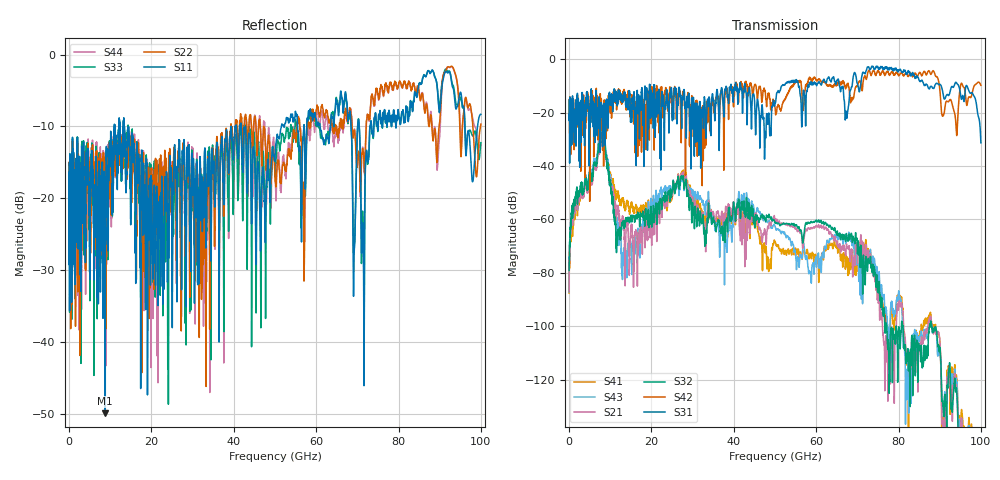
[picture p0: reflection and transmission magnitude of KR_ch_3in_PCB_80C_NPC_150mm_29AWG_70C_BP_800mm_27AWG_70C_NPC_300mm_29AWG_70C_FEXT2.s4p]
# GHz S RI R 45
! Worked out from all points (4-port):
!   4000 points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, 25 MHz to 100 GHz, reference 45 ohm
!   strongest paths, dB at 25 MHz, 25.02 GHz, 50.02 GHz, 75.03 GHz, 100 GHz:
!     S31: -20.7, -17.6, -16.4, -3.0, -31.3
!     S42: -20.7, -17.7, -18.0, -4.4, -9.7
!     S32: -79.1, -49.5, -61.3, -84.9, -155.0
!     S21: -86.8, -50.4, -60.1, -87.8, -157.8
!     S43: -87.1, -48.6, -62.6, -81.2, -149.6
!     S41: -87.6, -51.8, -68.5, -83.1, -149.4
!   lowest |S11| = -50.0 dB at 8.8 GHz (marker M1), VSWR 1.01, Z = 44.8 - j0.241 ohm
!   |S11| at or under -10 dB: start of sweep to 11.02 GHz; 13.41 GHz to 39.39 GHz (25.99 GHz wide, 98.4 % of centre); 42.84 GHz to 51.56 GHz (8.725 GHz wide, 18.5 % of centre)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
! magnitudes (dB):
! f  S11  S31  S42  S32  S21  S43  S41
! 25 MHz  -16.4  -20.7  -20.7  -79.1  -86.8  -87.1  -87.6
! 8.8 GHz  -50.0  -23.5  -15.5  -32.8  -34.0  -31.6  -32.8
! 13.22 GHz  -9.3  -13.6  -11.9  -61.5  -60.5  -73.4  -53.2
! 27.4 GHz  -19.2  -18.9  -16.4  -44.4  -43.2  -45.2  -42.6
! 48.55 GHz  -17.3  -20.9  -12.7  -58.0  -62.0  -60.4  -78.4
! 74.9 GHz  -10.1  -2.6  -4.4  -86.6  -90.2  -81.9  -84.4
! 100 GHz  -8.3  -31.3  -9.7  -155.0  -157.8  -149.6  -149.4
